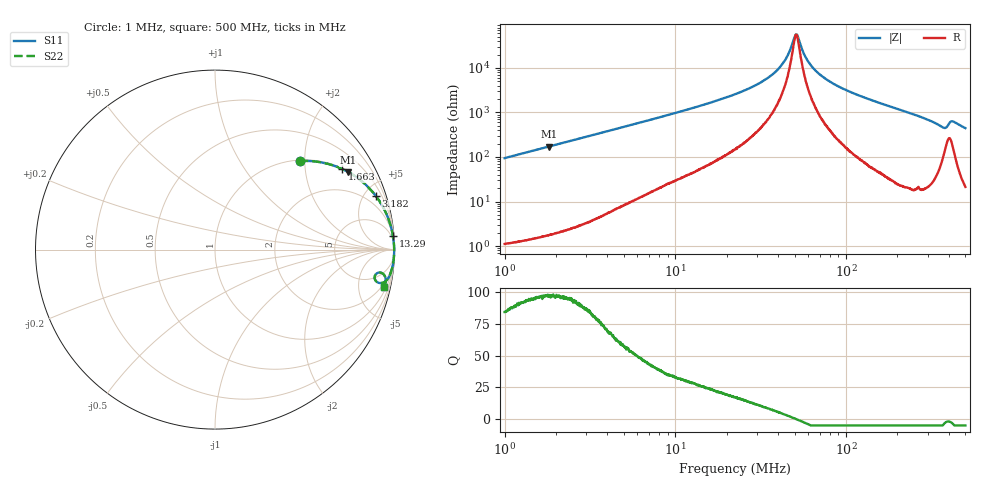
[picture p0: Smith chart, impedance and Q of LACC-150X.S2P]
!s-Parameter Generated by FASTRON Sdn. Bhd.
!FASTRON P/N : LACC-150X
!Keysight Technologies,E4991B,MY54100416,A.01.15
!Date: Wed Mar 18 09:30:17 2026
!Version  : Rev00 Wed Mar 18 09:30:17 2026
!Data & Calibration Information:
!PortZ  Port1:50+j0  Port2:50+j0
!When reading, reference impedance value at option line is always used.
!Remarks : This data is being provided solely for informational purposes.
!Freq	S11	S21	S12	S22
# Hz S dB R 50
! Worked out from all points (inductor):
!   1601 points, 1 MHz to 500 MHz, reference 50 ohm
!   read as one part in series: L = 15 uH near 1.032 MHz
!   highest Q = 97.6 at 1.812 MHz (marker M1), where L = 15 uH
!   self-resonance near 50.94 MHz
!   S11 on the Smith chart (normalised r, x): 1 MHz: 1.02, +1.89; 1.663 MHz: 1.03, +3.14; 3.182 MHz: 1.07, +6.03; 13.29 MHz: 2, +27; 500 MHz: 1.43, -8.90
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1000000  -3.32 46.3  -2.82 -43.0  -2.82 -43.0  -3.32 46.3
1663329  -1.52 32.3  -5.44 -57.1  -5.44 -57.1  -1.52 32.3
1811711  -1.31 30.1  -5.98 -59.3  -5.98 -59.3  -1.31 30.1
2820919  -0.60 20.5  -9.13 -68.9  -9.13 -68.9  -0.60 20.5
3181875  -0.48 18.3  -10.07 -71.0  -10.07 -71.0  -0.48 18.3
7957584  -0.10 7.4  -17.79 -81.1  -17.79 -81.1  -0.10 7.4
1.328759e7  -0.05 4.3  -22.54 -83.6  -22.54 -83.6  -0.05 4.3
2.236068e7  -0.03 2.2  -28.21 -84.4  -28.21 -84.4  -0.03 2.2
3.110769e7  -0.02 1.2  -33.20 -83.4  -33.20 -83.4  -0.02 1.2
3.88167e7  -0.02 0.7  -38.49 -80.1  -38.49 -80.1  -0.02 0.7
4.446912e7  -0.02 0.3  -44.25 -72.7  -44.25 -72.7  -0.02 0.3
5.074715e7  -0.02 0.0  -54.88 -8.2  -54.88 -8.2  -0.02 0.0
5.214584e7  -0.02 -0.1  -54.09 27.4  -54.09 27.4  -0.02 -0.1
5.746337e7  -0.02 -0.3  -45.40 70.5  -45.40 70.5  -0.02 -0.3
6.307767e7  -0.02 -0.5  -40.58 78.9  -40.58 78.9  -0.02 -0.5
7.282648e7  -0.02 -0.9  -36.10 83.2  -36.10 83.2  -0.02 -0.9
8.947314e7  -0.02 -1.5  -31.86 85.0  -31.86 85.0  -0.02 -1.5
1.77937e8  -0.04 -4.1  -22.92 84.6  -22.92 84.6  -0.04 -4.1
3.664557e8  -0.51 -11.4  -13.93 68.0  -13.93 68.0  -0.51 -11.4
3.82452e8  -0.82 -10.9  -13.90 58.3  -13.90 58.3  -0.82 -10.9
4.181909e8  -0.49 -8.1  -16.55 64.2  -16.55 64.2  -0.49 -8.1
5e8  -0.30 -12.5  -13.28 74.8  -13.28 74.8  -0.30 -12.5
